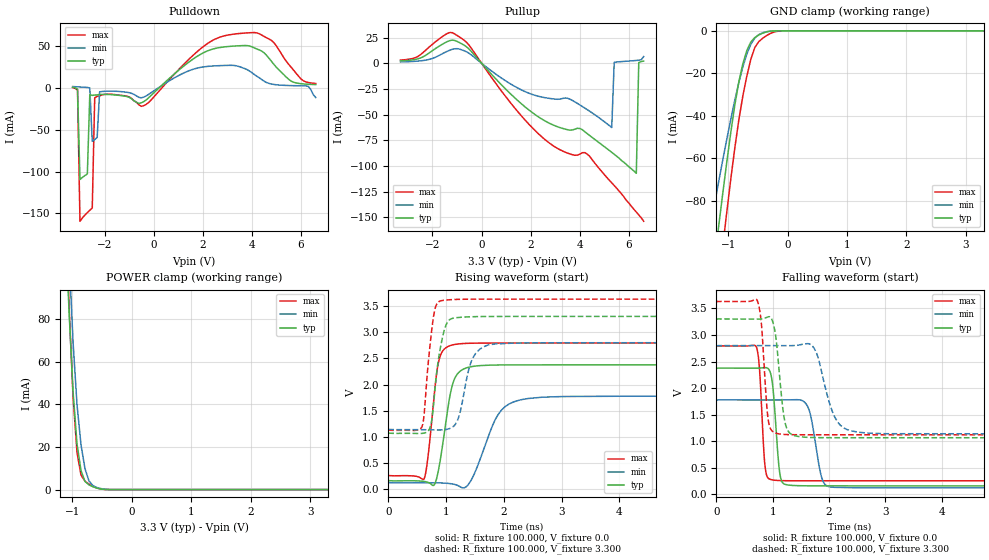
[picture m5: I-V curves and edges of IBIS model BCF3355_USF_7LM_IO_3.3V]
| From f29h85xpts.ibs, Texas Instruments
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|BCF3355_USF_7LM_IO_3.3V;
|   Model BCF3355_USF_7LM_IO_3.3V
[Model]   BCF3355_USF_7LM_IO_3.3V
Model_type   I/O
Polarity   Non-Inverting
Enable   Active-Low
Vinl =   0.800V
Vinh =   2.000V
Vmeas =  1.650V
Cref =   15.000pF
Vref =   0.0V
|   typ   min   max
C_comp   1.818pF   1.815pF   1.869pF
[Model Spec]
Vinh   2.000V   2.000V   2.000V
Vinl   0.800V   0.800V   0.800V
[Temperature Range]   25   155   -40
[Voltage Range]   3.300V   2.800V   3.630V
[Pullup Reference]   3.300V   2.800V   3.630V
[Pulldown Reference]   0.0V   0.0V   0.0V
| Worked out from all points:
|   slope of the pulldown table from 0 to 0.495 V, typ, clamps not added: 36.2 ohm
|   slope of the pullup table from 0 to 0.495 V, typ, clamps not added: 37.8 ohm
|   GND clamp passes 1 mA (typ) near -0.41 V on its own axis
|   POWER clamp passes 1 mA (typ) near -0.62 V on its own axis
|   rising waveform, R_fixture 100.000, V_fixture 0.0: 20-80 % time 190ps typ, 366ps min, 145ps max; typ from 0.161 V to 2.38 V
|   rising waveform, R_fixture 100.000, V_fixture 3.300: 20-80 % time 156ps typ, 206ps min, 127ps max; typ from 1.07 V to 3.3 V
|   falling waveform, R_fixture 100.000, V_fixture 0.0: 20-80 % time 92.8ps typ, 158ps min, 75ps max; typ from 2.38 V to 0.16 V
|   falling waveform, R_fixture 100.000, V_fixture 3.300: 20-80 % time 125ps typ, 261ps min, 93.1ps max; typ from 3.3 V to 1.07 V
[Pulldown]
|Voltage   I(typ)   I(min)   I(max)
-3.3V     834.9uA    1.653mA    502uA
-3.1V     -1.312mA   1.306mA    -2.259mA
-3V       -109.5mA   1.133mA    -159.5mA
-2.7V     -102.9mA   572uA      -149.1mA
-2.6V     -8.166mA   27.9uA     -146.3mA
-2.5V     -8.923mA   -63.85mA   -143.7mA
-2.4V     -8.498mA   -61.79mA   -11.86mA
-2.3V     -8.358mA   -59.2mA    -10.06mA
-2.2V     -7.913mA   -4.659mA   -9.515mA
-400mV    -16.32mA   -10.97mA   -21.15mA
3.9V      50.14mA    20.23mA    65.97mA
6.6V      3.99mA     -11.46mA   5.342mA
[Pullup]
|Voltage   I(typ)   I(min)   I(max)
-3.3V     2.306mA    1.297mA    3.095mA
-1.1V     22.26mA    14.1mA     28.64mA
-500mV    13.58mA    9.568mA    17.35mA
1.1V      -27.9mA    -18.92mA   -36.03mA
2.3V      -51.89mA   -32mA      -68.25mA
3.4V      -64.03mA   -33.73mA   -86.42mA
4.3V      -68.39mA   -45.06mA   -88.33mA
5.3V      -86.63mA   -62.47mA   -116.3mA
5.4V      -88.51mA   854.1uA    -118.9mA
6.3V      -107mA     2.75mA     -144.7mA
6.4V      661.5uA    3.003mA    -147.5mA
6.6V      2.129mA    6.529mA    -153.7mA
[GND_clamp]
|Voltage   I(typ)   I(min)   I(max)
-3.3V     -609.2mA   -407.2mA   -664.4mA
-1.29V    -122mA     -90.72mA   -150.4mA
-1.156V   -91.06mA   -70.38mA   -117.2mA
-1.089V   -76.03mA   -60.47mA   -100.9mA
-1.022V   -61.45mA   -50.81mA   -84.96mA
-888mV    -34.91mA   -32.58mA   -55.02mA
-821mV    -24.08mA   -24.35mA   -41.94mA
-687mV    -9.365mA   -10.96mA   -21.45mA
-620mV    -5.289mA   -6.391mA   -13.52mA
-486mV    -1.98mA    -1.783mA   -5.123mA
-84mV     -382.5nA   -1.742uA   -22.33uA
3.3V      0A         0A         0A
[POWER_clamp]
|Voltage   I(typ)   I(min)   I(max)
-3.3V     2.006A     2.24A      2.189A
-1.122V   128.4mA    157.6mA    136.9mA
-1.055V   83.34mA    109.6mA    86.06mA
-988mV    45.96mA    69.27mA    43.45mA
-921mV    21.31mA    39.69mA    17.29mA
-854mV    8.923mA    20.94mA    6.8mA
-787mV    3.841mA    9.787mA    3.88mA
-720mV    2.21mA     4.075mA    2.589mA
-653mV    1.325mA    1.86mA     1.547mA
-586mV    682.2uA    961.2uA    740.8uA
-385mV    14.58uA    59.34uA    8.752uA
3.3V      0A         0A         0A
[Ramp]
| variable   typ   min   max
dV/dt_r   1.329/0.189n   0.992/0.365n   1.521/0.145n
dV/dt_f   1.339/0.125n   0.997/0.261n   1.504/92.866p
R_load = 100.000
[Rising Waveform]
R_fixture= 100.000
V_fixture= 0.0
V_fixture_min= 0.0
V_fixture_max= 0.0
|time   V(typ)   V(min)   V(max)
0s        160.5mV    123.2mV    256.3mV
618ps     152.3mV    126.3mV    200mV
685ps     134.8mV    126.3mV    606.1mV
788ps     79.5mV     125.7mV    1.722V
874ps     400.9mV    123.9mV    2.45V
1.126ns   2.051V     99.93mV    2.758V
1.431ns   2.339V     169.5mV    2.787V
1.956ns   2.373V     1.509V     2.791V
2.416ns   2.374V     1.733V     2.791V
10ns      2.375V     1.777V     2.791V
[Rising Waveform]
R_fixture= 100.000
V_fixture= 3.300
V_fixture_min= 2.800
V_fixture_max= 3.630
|time   V(typ)   V(min)   V(max)
0s        1.066V     1.138V     1.122V
582ps     1.068V     1.139V     1.194V
718ps     1.167V     1.136V     2.709V
782ps     1.606V     1.134V     3.294V
916ps     2.786V     1.134V     3.598V
1.016ns   3.175V     1.146V     3.612V
1.194ns   3.276V     1.307V     3.623V
1.441ns   3.292V     2.452V     3.627V
1.729ns   3.297V     2.754V     3.628V
10ns      3.299V     2.799V     3.628V
[Falling Waveform]
R_fixture= 100.000
V_fixture= 0.0
V_fixture_min= 0.0
V_fixture_max= 0.0
|time   V(typ)   V(min)   V(max)
0s        2.375V     1.777V     2.791V
714ps     2.375V     1.776V     2.766V
866ps     2.385V     1.776V     517.1mV
971ps     2.247V     1.776V     279.2mV
1.125ns   408.3mV    1.776V     260.3mV
1.257ns   178.7mV    1.778V     257.2mV
1.621ns   161.8mV    1.654V     256.3mV
1.866ns   161mV      329.7mV    256.2mV
2.012ns   160.8mV    141.5mV    256.2mV
10ns      160.5mV    123.2mV    256.2mV
[Falling Waveform]
R_fixture= 100.000
V_fixture= 3.300
V_fixture_min= 2.800
V_fixture_max= 3.630
|time   V(typ)   V(min)   V(max)
0s        3.298V     2.799V     3.628V
730ps     3.298V     2.799V     3.639V
802ps     3.301V     2.799V     3.184V
922ps     3.341V     2.799V     1.398V
1.082ns   2.71V      2.799V     1.145V
1.221ns   1.346V     2.799V     1.127V
1.445ns   1.091V     2.806V     1.122V
1.733ns   1.069V     2.751V     1.122V
2.522ns   1.066V     1.169V     1.122V
10ns      1.066V     1.138V     1.122V
